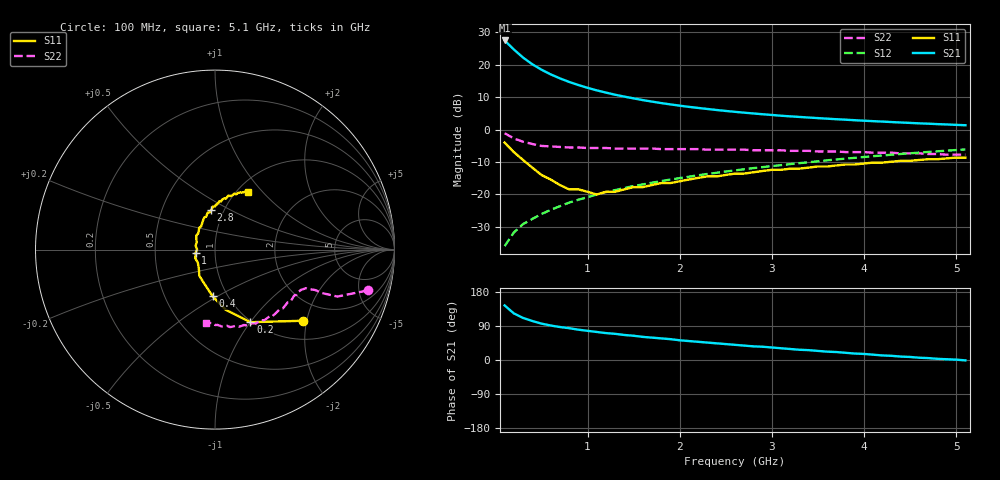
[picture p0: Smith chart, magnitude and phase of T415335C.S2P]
!AT-41533
!S and NOISE PARAMETERS at Vce=5V  Ic=10mA.  LAST UPDATED 01-25-95
# ghz s ma r 50
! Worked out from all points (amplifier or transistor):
!   51 points, 100 MHz to 5.1 GHz, reference 50 ohm
!   highest |S21| = 27.4 dB at 100 MHz (marker M1)
!   |S21| within 3 dB of that: start of sweep to 208.9 MHz
!   unconditionally stable (mu >= 1): 671.4 MHz to 2.178 GHz
!   at 900 MHz: K = 1.02, MAG = 16.7 dB, |S12| = -21.6 dB
!   at 2.6 GHz: K = 0.97, MSG = 9.0 dB, |S12| = -12.6 dB
!   at 5.1 GHz: K = 0.86, MSG = 3.7 dB, |S12| = -6.1 dB
!   lowest NFmin = 0.80 dB at 100 MHz
!   S11 on the Smith chart (normalised r, x): 100 MHz: 1.44, -1.90; 200 MHz: 0.99, -1.00; 400 MHz: 0.85, -0.47; 1 GHz: 0.80, -0.03; 2.8 GHz: 0.87, +0.40; 5.1 GHz: 1.13, +0.84
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0.1  0.63 -39.0  23.58 144.0  0.016 73.0  0.88 -15.0
0.2  0.45 -64.0  17.12 123.0  0.026 68.0  0.73 -21.0
0.3  0.34 -80.0  12.85 111.0  0.035 68.0  0.65 -22.0
0.4  0.26 -93.0  10.15 103.0  0.042 69.0  0.6 -22.0
0.5  0.2 -107.0  8.358 96.0  0.05 69.0  0.56 -23.0
0.6  0.17 -121.0  7.081 91.0  0.058 70.0  0.55 -23.0
0.7  0.14 -130.0  6.145 87.0  0.066 70.0  0.54 -24.0
0.8  0.12 -143.0  5.418 84.0  0.075 71.0  0.53 -25.0
0.9  0.12 -156.0  4.855 80.0  0.083 71.0  0.53 -25.0
1  0.11 -170.0  4.393 77.0  0.091 70.0  0.52 -27.0
1.1  0.1 179.0  4.016 74.0  0.1 70.0  0.52 -27.0
1.2  0.11 169.0  3.71 71.0  0.109 70.0  0.52 -29.0
1.3  0.11 158.0  3.438 69.0  0.117 70.0  0.51 -30.0
1.4  0.12 150.0  3.216 66.0  0.126 69.0  0.51 -31.0
1.6  0.13 136.0  2.842 61.0  0.143 68.0  0.51 -33.0
1.8  0.15 126.0  2.558 57.0  0.161 67.0  0.5 -36.0
2.1  0.17 114.0  2.237 50.0  0.188 64.0  0.5 -40.0
2.6  0.21 101.0  1.876 40.0  0.235 60.0  0.49 -47.0
2.8  0.22 96.0  1.77 36.0  0.255 58.0  0.48 -50.0
3.5  0.27 85.0  1.501 24.0  0.325 52.0  0.46 -63.0
4.3  0.32 72.0  1.305 11.0  0.41 43.0  0.44 -79.0
5.1  0.37 60.0  1.166 -1.0  0.494 33.0  0.41 -97.0
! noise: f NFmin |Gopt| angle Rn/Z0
0.1  0.8  0.35  8  0.16
0.9  1.1  0.16  109  0.11
1.8  1.5  0.35  -147  0.1
2.4  1.7  0.51  -117  0.19
